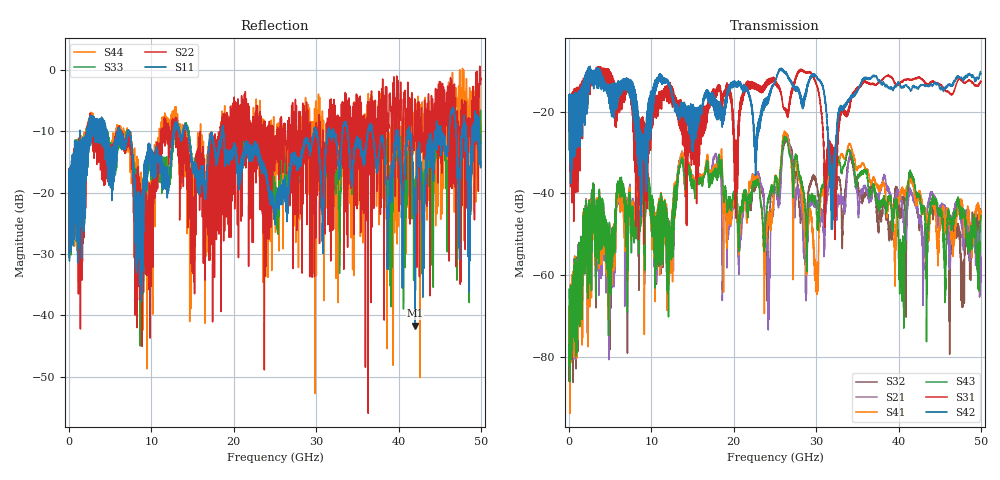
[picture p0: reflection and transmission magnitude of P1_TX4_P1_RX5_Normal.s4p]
!Keysight Technologies,N5225B,MY57041031,A.13.20.10
!Date: Friday, May 31, 2019 11:20:50
!Correction: S11(Full 4 Port(1,2,3,4))
!S12(Full 4 Port(1,2,3,4))
!S13(Full 4 Port(1,2,3,4))
!S14(Full 4 Port(1,2,3,4))
!S21(Full 4 Port(1,2,3,4))
!S22(Full 4 Port(1,2,3,4))
!S23(Full 4 Port(1,2,3,4))
!S24(Full 4 Port(1,2,3,4))
!S31(Full 4 Port(1,2,3,4))
!S32(Full 4 Port(1,2,3,4))
!S33(Full 4 Port(1,2,3,4))
!S34(Full 4 Port(1,2,3,4))
!S41(Full 4 Port(1,2,3,4))
!S42(Full 4 Port(1,2,3,4))
!S43(Full 4 Port(1,2,3,4))
!S44(Full 4 Port(1,2,3,4))
!S4P File: Measurements: <S11,S12,S13,S14>,
!<S21,S22,S23,S24>,
!<S31,S32,S33,S34>,
!<S41,S42,S43,S44>:
# Hz S  dB  R 50.0
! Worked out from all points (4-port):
!   5000 points, 10 MHz to 50 GHz, reference 50 ohm
!   strongest paths, dB at 10 MHz, 12.51 GHz, 25.01 GHz, 37.51 GHz, 50 GHz:
!     S42: -19.5, -15.6, -12.9, -12.3, -10.7
!     S31: -19.7, -17.6, -12.9, -13.1, -12.6
!     S43: -63.4, -46.4, -36.4, -41.8, -45.4
!     S41: -67.5, -47.1, -36.0, -37.9, -44.7
!     S21: -72.7, -46.0, -38.7, -41.4, -57.9
!     S32: -71.1, -45.9, -38.6, -48.1, -44.9
!   lowest |S11| = -41.7 dB at 42 GHz (marker M1), VSWR 1.02, Z = 49.3 + j0.442 ohm
!   |S11| at or under -10 dB: 7.336 GHz to 12.7 GHz (5.362 GHz wide, 53.5 % of centre); 14.41 GHz to 18.57 GHz (4.158 GHz wide, 25.2 % of centre); 18.74 GHz to 29.76 GHz (11.02 GHz wide, 45.4 % of centre)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
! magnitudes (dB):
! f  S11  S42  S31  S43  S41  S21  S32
! 10 MHz  -19.5  -19.5  -19.7  -63.4  -67.5  -72.7  -71.1
! 13.64 GHz  -10.8  -19.1  -24.1  -31.7  -30.5  -30.1  -31.1
! 24.24 GHz  -19.2  -15.9  -12.1  -40.8  -44.9  -69.1  -47.4
! 26.34 GHz  -20.2  -10.3  -19.5  -26.6  -25.4  -26.3  -26.8
! 30.03 GHz  -9.8  -11.5  -13.3  -42.7  -59.4  -42.0  -37.9
! 42 GHz  -41.7  -13.8  -11.9  -38.1  -40.8  -42.0  -38.9
! 50 GHz  -12.0  -10.7  -12.6  -45.4  -44.7  -57.9  -44.9
